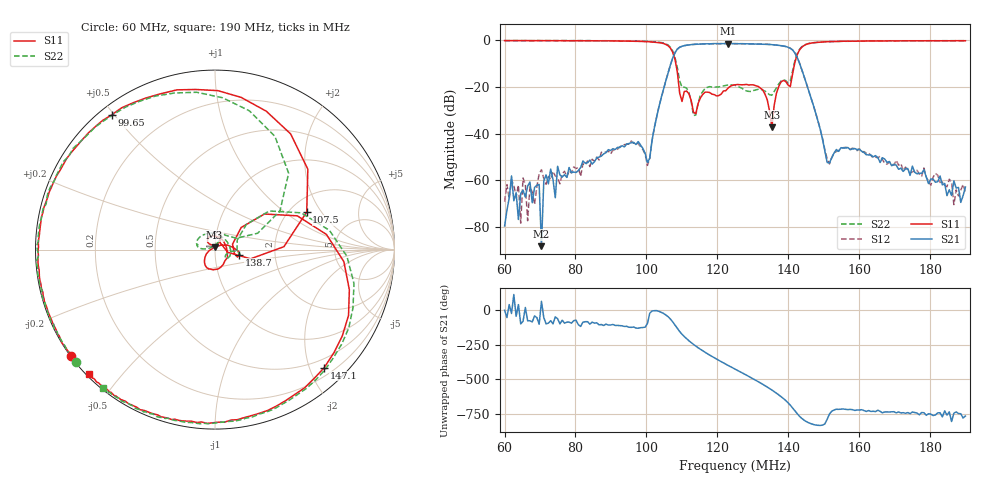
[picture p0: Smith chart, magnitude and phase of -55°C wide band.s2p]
!Agilent Technologies,E8362C,SG49020144,A.09.33.09
!Agilent E8362C: A.09.33.09
!Date: Friday, October 10, 2025 09:18:03
!Correction: S11(Full 2 Port(1,2))
!S21(Full 2 Port(1,2))
!S12(Full 2 Port(1,2))
!S22(Full 2 Port(1,2))
!S2P File: Measurements: S11, S21, S12, S22:
# Hz S  dB  R 50
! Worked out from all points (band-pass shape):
!   201 points, 60 MHz to 190 MHz, reference 50 ohm
!   highest |S21| = -1.29 dB at 123 MHz (marker M1); lowest = -88.4 dB at 70.4 MHz (marker M2)
!   |S21| within 3 dB of the highest: 108.5 MHz to 141.4 MHz (32.89 MHz wide, 26.3 % of centre)
!   lowest |S11| = -37.3 dB at 135.4 MHz (marker M3), VSWR 1.03, Z = 49.8 + j1.35 ohm
!   |S11| at or under -10 dB: 108.3 MHz to 141.8 MHz (33.52 MHz wide, 26.8 % of centre)
!   |S22| runs from -32.3 to 0.0 dB; largest |S21 - S12| = 0.0087
!   S11 on the Smith chart (normalised r, x): 60 MHz: 0.00, -0.33; 99.65 MHz: 0.03, +0.49; 107.5 MHz: 2.46, +1.48; 138.7 MHz: 1.31, -0.08; 147.1 MHz: 0.34, -2.25; 190 MHz: 0.01, -0.41
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6e7  -0.03 -143.7  -79.75 1.3  -69.31 40.6  -0.06 -141.0
6.195e7  -0.05 -146.6  -58.26 -22.7  -60.04 -14.4  -0.05 -143.8
6.455e7  -0.05 -150.1  -65.84 -98.6  -78.56 26.2  -0.06 -147.4
6.52e7  -0.07 -151.1  -64.37 -79.6  -59.11 -94.2  -0.06 -148.3
6.65e7  -0.07 -153.1  -62.60 -76.0  -77.49 31.6  -0.05 -150.0
6.975e7  -0.07 -158.2  -61.90 -101.1  -57.29 -94.1  -0.03 -154.3
7.04e7  -0.07 -159.2  -88.44 65.2  -55.55 -43.4  -0.09 -155.2
7.17e7  -0.08 -160.9  -57.80 -98.2  -61.85 -54.5  -0.04 -157.2
8.21e7  -0.14 -178.1  -51.81 -85.9  -52.95 -80.7  -0.05 -173.0
9.965e7  -0.48 127.5  -48.55 -121.7  -48.90 -122.1  -0.39 138.4
1.0355e8  -0.93 96.9  -28.50 -7.4  -28.39 -7.7  -0.74 111.4
1.0745e8  -5.16 22.3  -7.44 -84.6  -7.40 -84.3  -4.56 46.1
1.107e8  -21.94 71.0  -2.19 169.2  -2.22 169.1  -20.06 68.6
1.146e8  -27.05 135.0  -1.59 88.1  -1.56 88.2  -26.94 175.8
1.2305e8  -20.44 -61.1  -1.29 -40.1  -1.37 -39.9  -19.10 157.0
1.25e8  -19.09 -89.4  -1.36 -66.8  -1.35 -66.5  -19.25 135.6
1.354e8  -37.28 98.8  -1.77 141.3  -1.77 141.2  -23.54 -24.4
1.3865e8  -17.17 -11.7  -2.36 79.4  -2.43 79.3  -16.90 -10.3
1.471e8  -0.95 -47.2  -27.82 -109.2  -27.81 -109.6  -0.97 -42.6
1.51e8  -0.51 -71.8  -52.46 -71.6  -50.88 -75.1  -0.54 -66.9
1.6855e8  -0.13 -115.0  -52.03 -18.6  -52.23 -29.0  -0.13 -109.3
1.9e8  -0.10 -135.4  -63.04 -47.9  -65.30 -66.6  -0.08 -128.9
